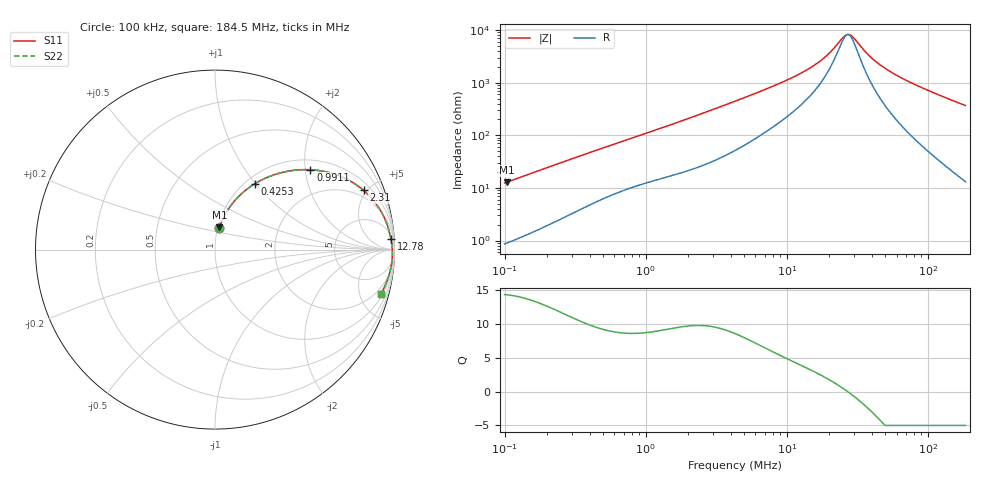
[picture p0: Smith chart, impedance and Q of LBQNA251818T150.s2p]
! LBQNA251818T150  S-PARAMETER MODEL  ( General Type )
! Model Generated by TAIYO YUDEN Corporation (http://www.ty-top.com)
! Version 1.0
! TAIYO YUDEN Control No. 191025NI43SB-FBB
! Copyright(c) 2019 TAIYO YUDEN CO.,LTD. All Rights Reserved.
! Product Description (link to TY-COMPAS)
! https://ds.yuden.co.jp/TYCOMPAS/or/detail?pn=LBQNA251818T150K&u=M
! Products Name : Inductors
! Characteristics :
!  Inductance : 15 uH , SRF(min) : 23 MHz , DC Resistance(max) : 0.416 Ohm
!  Rated Current : Saturation :180 mA , Temp Rise : 500 mA (20 degC)
!  Case Size : 2.5 x 1.8 / 0.098 x 0.071 [mm/inch] , Thickness : 1.8 / 0.071 [mm/inch]
!  (Conditions: Temperature = 25 degC , DC Bias Current/Voltage = 0A / 0V)
! External Node Assignments :
!  1  o---GGG---o  2
! GND o---------o GND
! Frequency Range : 0.1MHz  -  184.468258MHz  [ 402 STEP ]
# MHz S RI R 50
! Freq[MHz].  S11 Real  S11 Imag  S21 Real  S21 Imag  S12 Real  S12 Imag  S22 Real  S22 Imag
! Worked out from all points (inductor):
!   401 points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, 100 kHz to 184.5 MHz, reference 50 ohm
!   read as one part in series: L = 19.6 uH near 103.8 kHz
!   highest Q = 14.3 at 103.8 kHz (marker M1), where L = 19.7 uH
!   self-resonance near 27.03 MHz
!   S11 on the Smith chart (normalised r, x): 100 kHz: 1.02, +0.25; 425.3 kHz: 1.10, +0.99; 991.1 kHz: 1.24, +2.13; 2.31 MHz: 1.49, +4.76; 12.78 MHz: 9, +30; 184.5 MHz: 1.26, -7.34
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0.1  0.0232 0.1198  0.9768 -0.1198  0.9768 -0.1198  0.0232 0.1198
0.103832  0.0247 0.1241  0.9753 -0.1241  0.9753 -0.1241  0.0247 0.1241
0.204297  0.0737 0.2244  0.9263 -0.2244  0.9263 -0.2244  0.0737 0.2244
0.352405  0.1702 0.3305  0.8298 -0.3305  0.8298 -0.3305  0.1702 0.3305
0.425295  0.2204 0.366  0.7796 -0.366  0.7796 -0.366  0.2204 0.366
0.667798  0.3737 0.4297  0.6263 -0.4297  0.6263 -0.4297  0.3737 0.4297
0.991074  0.5319 0.4449  0.4681 -0.4449  0.4681 -0.4449  0.5319 0.4449
1.241892  0.6231 0.4323  0.3769 -0.4323  0.3769 -0.4323  0.6231 0.4323
2.309523  0.8274 0.3303  0.1726 -0.3303  0.1726 -0.3303  0.8274 0.3303
4.294977  0.9303 0.203  0.0697 -0.203  0.0697 -0.203  0.9303 0.203
8.138871  0.9691 0.107  0.0309 -0.107  0.0309 -0.107  0.9691 0.107
12.77966  0.9802 0.0604  0.0198 -0.0604  0.0198 -0.0604  0.9802 0.0604
15.13571  0.9829 0.0457  0.0171 -0.0457  0.0171 -0.0457  0.9829 0.0457
18.9662  0.9855 0.0274  0.0145 -0.0274  0.0145 -0.0274  0.9855 0.0274
25.14504  0.9877 0.00559  0.0123 -0.00559  0.0123 -0.00559  0.9877 0.00559
27.10888  0.988 -0.000219  0.012 0.000219  0.012 0.000219  0.988 -0.000219
29.2261  0.9883 -0.00607  0.0117 0.00607  0.0117 0.00607  0.9883 -0.00607
35.94047  0.9885 -0.0226  0.0115 0.0226  0.0115 0.0226  0.9885 -0.0226
40.99561  0.9882 -0.0337  0.0118 0.0337  0.0118 0.0337  0.9882 -0.0337
53.33896  0.9864 -0.0579  0.0136 0.0579  0.0136 0.0579  0.9864 -0.0579
90.29404  0.9757 -0.1194  0.0243 0.1194  0.0243 0.1194  0.9757 -0.1194
184.4683  0.9234 -0.2487  0.0766 0.2487  0.0766 0.2487  0.9234 -0.2487
